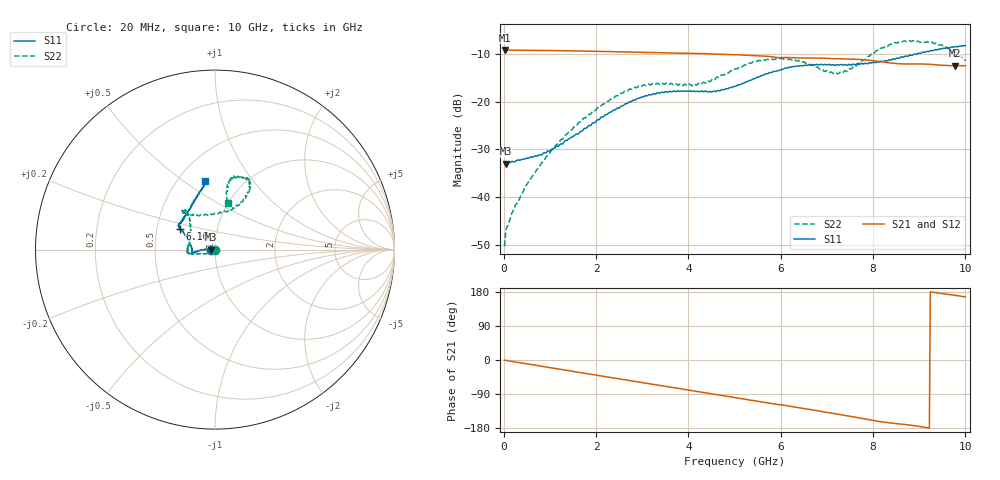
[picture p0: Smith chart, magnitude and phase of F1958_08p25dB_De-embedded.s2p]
! Integrated Device Technology
! Corporate Headquarters
! 6024 Silver Creek Valley Road
! San Jose, CA 95138  USA
! Phone:  1-408-284-8200
! Toll Free:  1-800-223-1366
! Webpage:  http://www.idt.com/
! Timing and RF Division
! 515 Groton Road, Suite 102
! Westford, MA 01886-6024
! Device:  F1958
! Description: 7-bit 0.25 dB Digital Step Attenuator
! Frequency:  0.001 -  6.000 GHz
! Package:  4x4 mm Thin QFN Plastic Package: 24 pin
! Ports:  2 RF, 12 DC
!  Pin  1  = D0
!  Pin  2  = VDD
!  Pin  3  = VMODE
!  Pin  4  = GND
!  Pin  5  = RF1  =  Port 1
!  Pin  6  = GND
!  Pin  7  = GND
!  Pin  8  = GND
!  Pin  9  = GND
!  Pin 10  = GND
!  Pin 11  = GND
!  Pin 12  = GND
!  Pin 13  = GND
!  Pin 14  = RF2  =  Port 2
!  Pin 15  = GND
!  Pin 16  = LE
!  Pin 17  = CLK
!  Pin 18  = DATA
!  Pin 19  = D6
!  Pin 20  = D5
!  Pin 21  = D4
!  Pin 22  = D3
!  Pin 23  = D2
!  Pin 24  = D1
! State:  33
! Atten State:  8.25 dB
! Voltage:  +3.30 Volts
! Current:  0.258 mA
! Data:  The device was measured on a F1958 evaluation board which has
!  individual transmission lines to the RF pins.  Data was collected
!  using a calibrated network analyzer.  The evaluation board was
!  de-embedded using Automatic Fixture Removal (AFR).
!  The reference plane is the edge of the package pin.
! Misc:
!  Action Tracker AT0419
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# GHz S dB R 50
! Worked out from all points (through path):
!   500 points, 20 MHz to 10 GHz, reference 50 ohm
!   highest |S21| = -9.16 dB at 20 MHz (marker M1); lowest = -12.5 dB at 9.78 GHz (marker M2)
!   group delay of S21, straight-line fit = 54.2 ps
!   lowest |S11| = -33.0 dB at 40 MHz (marker M3), VSWR 1.05, Z = 47.8 - j0.0784 ohm
!   |S11| at or under -10 dB: start of sweep to 8.948 GHz
!   |S22| runs from -50.3 to -7.2 dB; largest |S21 - S12| = 0.00094
!   S11 on the Smith chart (normalised r, x): 20 MHz: 0.96, -0.00; 6.16 GHz: 0.66, +0.16; 10 GHz: 0.68, +0.61
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0.02  -32.96 -178.1  -9.16 -0.5  -9.16 -0.5  -50.29 -137.4
0.04  -33.00 -177.9  -9.17 -0.9  -9.16 -0.9  -47.68 -133.2
0.08  -32.80 -179.4  -9.18 -1.8  -9.18 -1.8  -46.09 -127.9
0.2  -32.55 178.5  -9.20 -4.2  -9.20 -4.2  -42.97 -131.8
0.5  -31.85 174.3  -9.23 -10.1  -9.22 -10.1  -37.41 -134.6
1.02  -30.19 175.3  -9.27 -20.5  -9.27 -20.5  -30.37 -143.4
1.7  -26.16 179.2  -9.38 -33.9  -9.37 -33.9  -23.89 -159.1
2.58  -20.85 -174.7  -9.56 -51.3  -9.55 -51.3  -18.19 -169.1
3.36  -18.20 -170.5  -9.74 -66.7  -9.74 -66.8  -16.30 -174.6
4.22  -17.85 -174.0  -9.90 -83.5  -9.91 -83.6  -16.16 156.8
5.02  -16.79 165.6  -10.14 -99.4  -10.15 -99.4  -13.08 130.3
5.54  -14.76 154.4  -10.40 -109.7  -10.41 -109.7  -11.38 127.7
6.16  -12.86 149.2  -10.73 -121.2  -10.75 -121.2  -11.16 130.1
6.68  -12.25 146.1  -10.85 -131.3  -10.87 -131.3  -12.34 125.0
7.06  -12.20 143.1  -10.93 -139.7  -10.94 -139.5  -13.90 107.0
7.3  -12.19 140.5  -11.01 -144.3  -11.01 -144.2  -13.85 90.0
7.9  -11.92 129.2  -11.29 -157.3  -11.28 -157.4  -10.48 62.3
8.34  -11.26 119.7  -11.84 -165.7  -11.84 -165.8  -8.20 59.9
8.74  -10.50 112.0  -12.10 -170.9  -12.11 -170.9  -7.34 64.5
9.24  -9.30 102.8  -12.18 179.8  -12.19 179.8  -7.63 74.4
9.78  -8.44 98.4  -12.48 170.6  -12.50 170.6  -9.54 78.3
10  -8.27 98.0  -12.44 166.4  -12.48 166.5  -11.38 74.5
